DATA_BLOCK "IMAC_TANK_I/O"
TITLE =
AUTHOR : HottendU
FAMILY : IMAC
VERSION : 0.2


  STRUCT
   TANK_001_XTsub : REAL ;	//TANK - Instance 001 : Temperature Substitution Value
   TANK_001_XDensity : REAL ;	//                      Density of Medium in the Tank
   TANK_001_XReftemp : REAL ;	//                      Reference Temperature for given density
   TANK_001_XVEC : REAL ;	//                      Volume Expansion Coefficient
   TANK_001_YVolume : REAL ;	//                      Computed Volume in Tank (m3)
   TANK_001_YMass : REAL ;	//                      Computed Mass of Medium in Tank (tons)
   TANK_001_YLevel : REAL ;	//                      Computed Level of Medium in Tank (m)
   TANK_001_OSSTAT : WORD ;	//                      OS Status Word
   TANK_001_OSALARM : WORD ;	//                      OS Alarm Word
   TANK_002_XTsub : REAL ;	//TANK - Instance 002 : Temperature Substitution Value
   TANK_002_XDensity : REAL ;	//                      Density of Medium in the Tank
   TANK_002_XReftemp : REAL ;	//                      Reference Temperature for given density
   TANK_002_XVEC : REAL ;	//                      Volume Expansion Coefficient
   TANK_002_YVolume : REAL ;	//                      Computed Volume in Tank (m3)
   TANK_002_YMass : REAL ;	//                      Computed Mass of Medium in Tank (tons)
   TANK_002_YLevel : REAL ;	//                      Computed Level of Medium in Tank (m)
   TANK_002_OSSTAT : WORD ;	//                      OS Status Word
   TANK_002_OSALARM : WORD ;	//                      OS Alarm Word
   TANK_003_XTsub : REAL ;	//TANK - Instance 003 : Temperature Substitution Value
   TANK_003_XDensity : REAL ;	//                      Density of Medium in the Tank
   TANK_003_XReftemp : REAL ;	//                      Reference Temperature for given density
   TANK_003_XVEC : REAL ;	//                      Volume Expansion Coefficient
   TANK_003_YVolume : REAL ;	//                      Computed Volume in Tank (m3)
   TANK_003_YMass : REAL ;	//                      Computed Mass of Medium in Tank (tons)
   TANK_003_YLevel : REAL ;	//                      Computed Level of Medium in Tank (m)
   TANK_003_OSSTAT : WORD ;	//                      OS Status Word
   TANK_003_OSALARM : WORD ;	//                      OS Alarm Word
   TANK_004_XTsub : REAL ;	//TANK - Instance 004 : Temperature Substitution Value
   TANK_004_XDensity : REAL ;	//                      Density of Medium in the Tank
   TANK_004_XReftemp : REAL ;	//                      Reference Temperature for given density
   TANK_004_XVEC : REAL ;	//                      Volume Expansion Coefficient
   TANK_004_YVolume : REAL ;	//                      Computed Volume in Tank (m3)
   TANK_004_YMass : REAL ;	//                      Computed Mass of Medium in Tank (tons)
   TANK_004_YLevel : REAL ;	//                      Computed Level of Medium in Tank (m)
   TANK_004_OSSTAT : WORD ;	//                      OS Status Word
   TANK_004_OSALARM : WORD ;	//                      OS Alarm Word
   TANK_005_XTsub : REAL ;	//TANK - Instance 005 : Temperature Substitution Value
   TANK_005_XDensity : REAL ;	//                      Density of Medium in the Tank
   TANK_005_XReftemp : REAL ;	//                      Reference Temperature for given density
   TANK_005_XVEC : REAL ;	//                      Volume Expansion Coefficient
   TANK_005_YVolume : REAL ;	//                      Computed Volume in Tank (m3)
   TANK_005_YMass : REAL ;	//                      Computed Mass of Medium in Tank (tons)
   TANK_005_YLevel : REAL ;	//                      Computed Level of Medium in Tank (m)
   TANK_005_OSSTAT : WORD ;	//                      OS Status Word
   TANK_005_OSALARM : WORD ;	//                      OS Alarm Word
   TANK_006_XTsub : REAL ;	//TANK - Instance 006 : Temperature Substitution Value
   TANK_006_XDensity : REAL ;	//                      Density of Medium in the Tank
   TANK_006_XReftemp : REAL ;	//                      Reference Temperature for given density
   TANK_006_XVEC : REAL ;	//                      Volume Expansion Coefficient
   TANK_006_YVolume : REAL ;	//                      Computed Volume in Tank (m3)
   TANK_006_YMass : REAL ;	//                      Computed Mass of Medium in Tank (tons)
   TANK_006_YLevel : REAL ;	//                      Computed Level of Medium in Tank (m)
   TANK_006_OSSTAT : WORD ;	//                      OS Status Word
   TANK_006_OSALARM : WORD ;	//                      OS Alarm Word
   TANK_007_XTsub : REAL ;	//TANK - Instance 007 : Temperature Substitution Value
   TANK_007_XDensity : REAL ;	//                      Density of Medium in the Tank
   TANK_007_XReftemp : REAL ;	//                      Reference Temperature for given density
   TANK_007_XVEC : REAL ;	//                      Volume Expansion Coefficient
   TANK_007_YVolume : REAL ;	//                      Computed Volume in Tank (m3)
   TANK_007_YMass : REAL ;	//                      Computed Mass of Medium in Tank (tons)
   TANK_007_YLevel : REAL ;	//                      Computed Level of Medium in Tank (m)
   TANK_007_OSSTAT : WORD ;	//                      OS Status Word
   TANK_007_OSALARM : WORD ;	//                      OS Alarm Word
   TANK_008_XTsub : REAL ;	//TANK - Instance 008 : Temperature Substitution Value
   TANK_008_XDensity : REAL ;	//                      Density of Medium in the Tank
   TANK_008_XReftemp : REAL ;	//                      Reference Temperature for given density
   TANK_008_XVEC : REAL ;	//                      Volume Expansion Coefficient
   TANK_008_YVolume : REAL ;	//                      Computed Volume in Tank (m3)
   TANK_008_YMass : REAL ;	//                      Computed Mass of Medium in Tank (tons)
   TANK_008_YLevel : REAL ;	//                      Computed Level of Medium in Tank (m)
   TANK_008_OSSTAT : WORD ;	//                      OS Status Word
   TANK_008_OSALARM : WORD ;	//                      OS Alarm Word
   TANK_009_XTsub : REAL ;	//TANK - Instance 010 : Temperature Substitution Value
   TANK_009_XDensity : REAL ;	//                      Density of Medium in the Tank
   TANK_009_XReftemp : REAL ;	//                      Reference Temperature for given density
   TANK_009_XVEC : REAL ;	//                      Volume Expansion Coefficient
   TANK_009_YVolume : REAL ;	//                      Computed Volume in Tank (m3)
   TANK_009_YMass : REAL ;	//                      Computed Mass of Medium in Tank (tons)
   TANK_009_YLevel : REAL ;	//                      Computed Level of Medium in Tank (m)
   TANK_009_OSSTAT : WORD ;	//                      OS Status Word
   TANK_009_OSALARM : WORD ;	//                      OS Alarm Word
   TANK_010_XTsub : REAL ;	//                      Temperature Substitution Value
   TANK_010_XDensity : REAL ;	//                      Density of Medium in the Tank
   TANK_010_XReftemp : REAL ;	//                      Reference Temperature for given density
   TANK_010_XVEC : REAL ;	//                      Volume Expansion Coefficient
   TANK_010_YVolume : REAL ;	//                      Computed Volume in Tank (m3)
   TANK_010_YMass : REAL ;	//                      Computed Mass of Medium in Tank (tons)
   TANK_010_YLevel : REAL ;	//                      Computed Level of Medium in Tank (m)
   TANK_010_OSSTAT : WORD ;	//                      OS Status Word
   TANK_010_OSALARM : WORD ;	//                      OS Alarm Word
  END_STRUCT ;
BEGIN
   TANK_001_XTsub := 0.000000e+000;
   TANK_001_XDensity := 0.000000e+000;
   TANK_001_XReftemp := 0.000000e+000;
   TANK_001_XVEC := 0.000000e+000;
   TANK_001_YVolume := 0.000000e+000;
   TANK_001_YMass := 0.000000e+000;
   TANK_001_YLevel := 0.000000e+000;
   TANK_001_OSSTAT := W#16#0;
   TANK_001_OSALARM := W#16#0;
   TANK_002_XTsub := 0.000000e+000;
   TANK_002_XDensity := 0.000000e+000;
   TANK_002_XReftemp := 0.000000e+000;
   TANK_002_XVEC := 0.000000e+000;
   TANK_002_YVolume := 0.000000e+000;
   TANK_002_YMass := 0.000000e+000;
   TANK_002_YLevel := 0.000000e+000;
   TANK_002_OSSTAT := W#16#0;
   TANK_002_OSALARM := W#16#0;
   TANK_003_XTsub := 0.000000e+000;
   TANK_003_XDensity := 0.000000e+000;
   TANK_003_XReftemp := 0.000000e+000;
   TANK_003_XVEC := 0.000000e+000;
   TANK_003_YVolume := 0.000000e+000;
   TANK_003_YMass := 0.000000e+000;
   TANK_003_YLevel := 0.000000e+000;
   TANK_003_OSSTAT := W#16#0;
   TANK_003_OSALARM := W#16#0;
   TANK_004_XTsub := 0.000000e+000;
   TANK_004_XDensity := 0.000000e+000;
   TANK_004_XReftemp := 0.000000e+000;
   TANK_004_XVEC := 0.000000e+000;
   TANK_004_YVolume := 0.000000e+000;
   TANK_004_YMass := 0.000000e+000;
   TANK_004_YLevel := 0.000000e+000;
   TANK_004_OSSTAT := W#16#0;
   TANK_004_OSALARM := W#16#0;
   TANK_005_XTsub := 0.000000e+000;
   TANK_005_XDensity := 0.000000e+000;
   TANK_005_XReftemp := 0.000000e+000;
   TANK_005_XVEC := 0.000000e+000;
   TANK_005_YVolume := 0.000000e+000;
   TANK_005_YMass := 0.000000e+000;
   TANK_005_YLevel := 0.000000e+000;
   TANK_005_OSSTAT := W#16#0;
   TANK_005_OSALARM := W#16#0;
   TANK_006_XTsub := 0.000000e+000;
   TANK_006_XDensity := 0.000000e+000;
   TANK_006_XReftemp := 0.000000e+000;
   TANK_006_XVEC := 0.000000e+000;
   TANK_006_YVolume := 0.000000e+000;
   TANK_006_YMass := 0.000000e+000;
   TANK_006_YLevel := 0.000000e+000;
   TANK_006_OSSTAT := W#16#0;
   TANK_006_OSALARM := W#16#0;
   TANK_007_XTsub := 0.000000e+000;
   TANK_007_XDensity := 0.000000e+000;
   TANK_007_XReftemp := 0.000000e+000;
   TANK_007_XVEC := 0.000000e+000;
   TANK_007_YVolume := 0.000000e+000;
   TANK_007_YMass := 0.000000e+000;
   TANK_007_YLevel := 0.000000e+000;
   TANK_007_OSSTAT := W#16#0;
   TANK_007_OSALARM := W#16#0;
   TANK_008_XTsub := 0.000000e+000;
   TANK_008_XDensity := 0.000000e+000;
   TANK_008_XReftemp := 0.000000e+000;
   TANK_008_XVEC := 0.000000e+000;
   TANK_008_YVolume := 0.000000e+000;
   TANK_008_YMass := 0.000000e+000;
   TANK_008_YLevel := 0.000000e+000;
   TANK_008_OSSTAT := W#16#0;
   TANK_008_OSALARM := W#16#0;
   TANK_009_XTsub := 0.000000e+000;
   TANK_009_XDensity := 0.000000e+000;
   TANK_009_XReftemp := 0.000000e+000;
   TANK_009_XVEC := 0.000000e+000;
   TANK_009_YVolume := 0.000000e+000;
   TANK_009_YMass := 0.000000e+000;
   TANK_009_YLevel := 0.000000e+000;
   TANK_009_OSSTAT := W#16#0;
   TANK_009_OSALARM := W#16#0;
   TANK_010_XTsub := 0.000000e+000;
   TANK_010_XDensity := 0.000000e+000;
   TANK_010_XReftemp := 0.000000e+000;
   TANK_010_XVEC := 0.000000e+000;
   TANK_010_YVolume := 0.000000e+000;
   TANK_010_YMass := 0.000000e+000;
   TANK_010_YLevel := 0.000000e+000;
   TANK_010_OSSTAT := W#16#0;
   TANK_010_OSALARM := W#16#0;
END_DATA_BLOCK

